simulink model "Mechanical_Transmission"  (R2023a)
settings: Solver=VariableStepAuto  StartTime=0.0  StopTime=10.0  RelTol=1e-3
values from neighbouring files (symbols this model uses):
  R = 1    [Mechanical_Transmission_EQN.m]    (also in Mechanical_Transmission_SLX_m.m; Electrical_Transformer_EQN.m; Electrical_Transformer_SLX_m.m; Mechanical_system_EQN.m)
undefined symbols (not defined in the file or in its folder): mTr
libraries: fl_lib x15, nesl_utility x2

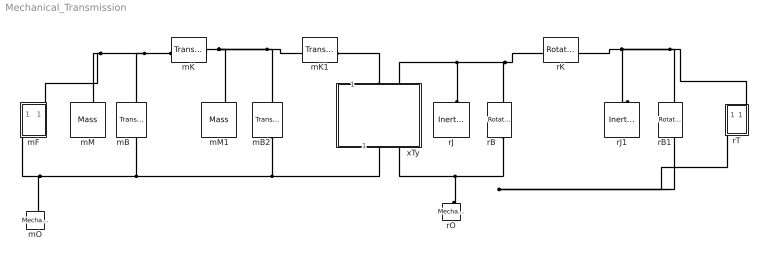
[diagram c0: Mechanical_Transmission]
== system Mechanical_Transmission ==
  mB : fl_lib/Mechanical/Translational Elements/Translational Damper  D=100 N*s/m  v_specify=off  v_priority=None  v=0 m/s  v_nominal_specify=off  v_nominal_unit=m/s  v_nominal_value=1  f_specify=off  f_priority=None  f=0 N  f_nominal_specify=off  f_nominal_unit=N  f_nominal_value=1
  mB2 : fl_lib/Mechanical/Translational Elements/Translational Damper  D=100 N*s/m  v_specify=off  v_priority=None  v=0 m/s  v_nominal_specify=off  v_nominal_unit=m/s  v_nominal_value=1  f_specify=off  f_priority=None  f=0 N  f_nominal_specify=off  f_nominal_unit=N  f_nominal_value=1
  mF : Subsystem  mask{mF='Fa'}
      mask prompts: mF "Output variable"
  mK : fl_lib/Mechanical/Translational Elements/Translational Spring  spr_rate=1000 N/m  v_specify=off  v_priority=None  v=0 m/s  v_nominal_specify=off  v_nominal_unit=m/s  v_nominal_value=1  f_specify=off  f_priority=None  f=0 N  f_nominal_specify=off  f_nominal_unit=N  f_nominal_value=1  x_specify=off  x_priority=High  x=0 m  x_nominal_specify=off  x_nominal_unit=m  x_nominal_value=1
  mK1 : fl_lib/Mechanical/Translational Elements/Translational Spring  spr_rate=1000 N/m  v_specify=off  v_priority=None  v=0 m/s  v_nominal_specify=off  v_nominal_unit=m/s  v_nominal_value=1  f_specify=off  f_priority=None  f=0 N  f_nominal_specify=off  f_nominal_unit=N  f_nominal_value=1  x_specify=off  x_priority=High  x=0 m  x_nominal_specify=off  x_nominal_unit=m  x_nominal_value=1
  mM : fl_lib/Mechanical/Translational Elements/Mass  mass=1 kg  num_ports=foundation.enum.numPorts2.one  v_specify=off  v_priority=High  v=0 m/s  v_nominal_specify=off  v_nominal_unit=m/s  v_nominal_value=1  f_specify=off  f_priority=None  f=0 N  f_nominal_specify=off  f_nominal_unit=N  f_nominal_value=1
  mM1 : fl_lib/Mechanical/Translational Elements/Mass  mass=1 kg  num_ports=foundation.enum.numPorts2.one  v_specify=off  v_priority=High  v=0 m/s  v_nominal_specify=off  v_nominal_unit=m/s  v_nominal_value=1  f_specify=off  f_priority=None  f=0 N  f_nominal_specify=off  f_nominal_unit=N  f_nominal_value=1
  mO : fl_lib/Mechanical/Translational Elements/Mechanical Translational Reference
  rB : fl_lib/Mechanical/Rotational Elements/Rotational Damper  D=0.001 N*m*s/rad  w_specify=off  w_priority=None  w=0 rad/s  w_nominal_specify=off  w_nominal_unit=rad/s  w_nominal_value=1  t_specify=off  t_priority=None  t=0 N*m  t_nominal_specify=off  t_nominal_unit=N*m  t_nominal_value=1
  rB1 : fl_lib/Mechanical/Rotational Elements/Rotational Damper  D=0.001 N*m*s/rad  w_specify=off  w_priority=None  w=0 rad/s  w_nominal_specify=off  w_nominal_unit=rad/s  w_nominal_value=1  t_specify=off  t_priority=None  t=0 N*m  t_nominal_specify=off  t_nominal_unit=N*m  t_nominal_value=1
  rJ : fl_lib/Mechanical/Rotational Elements/Inertia  inertia=0.01 kg*m^2  num_ports=foundation.enum.numPorts2.one  w_specify=off  w_priority=High  w=0 rad/s  w_nominal_specify=off  w_nominal_unit=rad/s  w_nominal_value=1  t_specify=off  t_priority=None  t=0 N*m  t_nominal_specify=off  t_nominal_unit=N*m  t_nominal_value=1
  rJ1 : fl_lib/Mechanical/Rotational Elements/Inertia  inertia=0.01 kg*m^2  num_ports=foundation.enum.numPorts2.one  w_specify=off  w_priority=High  w=0 rad/s  w_nominal_specify=off  w_nominal_unit=rad/s  w_nominal_value=1  t_specify=off  t_priority=None  t=0 N*m  t_nominal_specify=off  t_nominal_unit=N*m  t_nominal_value=1
  rK : fl_lib/Mechanical/Rotational Elements/Rotational Spring  spr_rate=10 N*m/rad  w_specify=off  w_priority=None  w=0 rad/s  w_nominal_specify=off  w_nominal_unit=rad/s  w_nominal_value=1  t_specify=off  t_priority=None  t=0 N*m  t_nominal_specify=off  t_nominal_unit=N*m  t_nominal_value=1  phi_specify=off  phi_priority=High  phi=0 rad  phi_nominal_specify=off  phi_nominal_unit=rad  phi_nominal_value=1
  rO : fl_lib/Mechanical/Rotational Elements/Mechanical Rotational Reference
  rT : Subsystem  mask{rT='Ta'}
      mask prompts: rT "Output variable"
  xTy : Subsystem  mask{Transformer_type=mTr, T_type=E1=K*E2, xTy=R}
      mask prompts: Transformer_type "Type of Transformer"; T_type "Type of relation"; xTy "Name of parameter K"
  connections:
  mB2/RConn1 -- xTy/RConn1 -- mB/RConn1 -- mF/RConn1 -- mO/LConn1
  mK/LConn1 -- mB/LConn1 -- mF/LConn1 -- mM/LConn1
  mK1/LConn1 -- mB2/LConn1 -- mM1/LConn1 -- mK/RConn1
  xTy/LConn1 -- mK1/RConn1
  rJ/LConn1 -- rK/LConn1 -- rB/LConn1 -- xTy/LConn2
  rB/RConn1 -- rT/RConn1 -- rB1/RConn1 -- xTy/RConn2 -- rO/LConn1
  rB1/LConn1 -- rT/LConn1 -- rK/RConn1 -- rJ1/LConn1

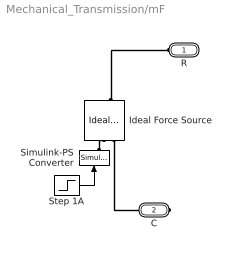
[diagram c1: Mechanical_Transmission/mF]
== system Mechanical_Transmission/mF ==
  Ideal Force Source : fl_lib/Mechanical/Mechanical Sources/Ideal Force Source
  Simulink-PS Converter : nesl_utility/Simulink-PS Converter  PhysicalDomain=network_engine_domain  SubClassName=ps_input  LeftPortType=input  RightPortType=output  PseudoPeriodic=off  Frequencies=[]  NoiseDistribution=none  NoiseParameters=[]  Unit=1  AffineConversion=off  FilteringAndDerivatives=zero  SimscapeFilterOrder=1  InputFilterTimeConstant=.001  UdotUserProvided=0
  Step 1A : Step  After=100  SampleTime=0
  R : PMIOPort  Side=Left
  C : PMIOPort  Port=2  Side=Right
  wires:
  Step 1A/1 -> Simulink-PS Converter/1
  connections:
  Simulink-PS Converter/RConn1 -- Ideal Force Source/RConn1
  Ideal Force Source/LConn1 -- R/RConn1
  Ideal Force Source/RConn2 -- C/RConn1

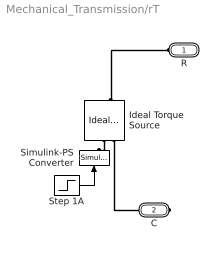
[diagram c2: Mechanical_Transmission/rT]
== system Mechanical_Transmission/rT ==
  Ideal Torque Source : fl_lib/Mechanical/Mechanical Sources/Ideal Torque Source
  Simulink-PS Converter : nesl_utility/Simulink-PS Converter  PhysicalDomain=network_engine_domain  SubClassName=ps_input  LeftPortType=input  RightPortType=output  PseudoPeriodic=off  Frequencies=[]  NoiseDistribution=none  NoiseParameters=[]  Unit=1  AffineConversion=off  FilteringAndDerivatives=zero  SimscapeFilterOrder=1  InputFilterTimeConstant=.001  UdotUserProvided=0
  Step 1A : Step  After=100  SampleTime=0
  R : PMIOPort  Side=Left
  C : PMIOPort  Port=2  Side=Right
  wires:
  Step 1A/1 -> Simulink-PS Converter/1
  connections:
  Ideal Torque Source/RConn2 -- C/RConn1
  Ideal Torque Source/LConn1 -- R/RConn1
  Ideal Torque Source/RConn1 -- Simulink-PS Converter/RConn1

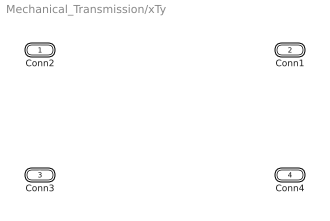
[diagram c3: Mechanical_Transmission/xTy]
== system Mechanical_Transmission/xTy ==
  Conn2 : PMIOPort  Side=Left
  Conn1 : PMIOPort  Port=2  Side=Left
  Conn3 : PMIOPort  Port=3  Side=Right
  Conn4 : PMIOPort  Port=4  Side=Right
